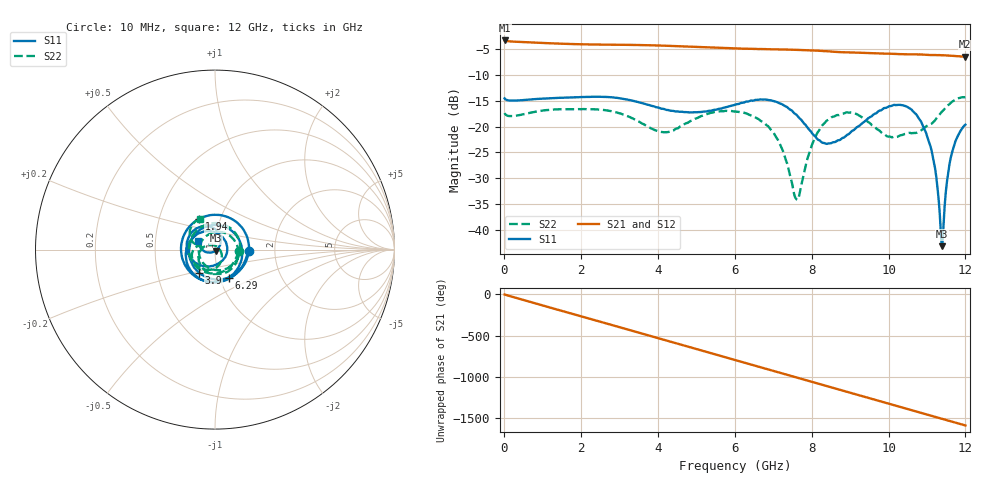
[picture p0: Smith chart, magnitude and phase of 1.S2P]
!Agilent Technologies,E5071C,MY46316741,A.11.02
!Date: Fri Apr 15 15:48:09 2022
!Data & Calibration Information:
!Freq	S11:SOLT2(ON)	S21:SOLT2(ON)	S12:SOLT2(ON)	S22:SOLT2(ON)
!PortZ  Port1:50+j0  Port2:50+j0
!Above PortZ is port z conversion or system Z0 setting when saving the data.
!When reading, reference impedance value at option line is always used.
# Hz S dB R 50
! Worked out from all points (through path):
!   1200 points, 10 MHz to 12 GHz, reference 50 ohm
!   highest |S21| = -3.32 dB at 10 MHz (marker M1); lowest = -6.5 dB at 11.99 GHz (marker M2)
!   group delay of S21, straight-line fit = 366 ps
!   lowest |S11| = -43.1 dB at 11.39 GHz (marker M3), VSWR 1.01, Z = 50.4 - j0.581 ohm
!   |S11| at or under -10 dB: start of sweep to end of sweep
!   |S22| runs from -34.2 to -14.3 dB; largest |S21 - S12| = 0.004
!   S11 on the Smith chart (normalised r, x): 10 MHz: 1.46, -0.03; 1.94 GHz: 0.79, +0.28; 3.9 GHz: 0.81, -0.22; 6.29 GHz: 1.11, -0.36; 12 GHz: 0.83, +0.08
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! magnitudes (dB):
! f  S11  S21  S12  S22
! 10 MHz  -14.5  -3.3  -3.3  -17.4
! 1.94 GHz  -14.3  -4.1  -4.0  -16.6
! 2.01 GHz  -14.3  -4.1  -4.1  -16.6
! 3.9 GHz  -16.1  -4.3  -4.3  -20.6
! 4.01 GHz  -16.3  -4.3  -4.3  -20.9
! 6.01 GHz  -15.7  -4.9  -4.9  -17.1
! 6.29 GHz  -15.2  -4.9  -4.9  -17.4
! 7.07 GHz  -15.2  -5.1  -5.0  -22.0
! 7.61 GHz  -17.7  -5.1  -5.1  -34.1
! 8.01 GHz  -21.3  -5.2  -5.2  -23.5
! 8.37 GHz  -23.3  -5.4  -5.4  -19.0
! 8.92 GHz  -21.6  -5.6  -5.6  -17.3
! 10.01 GHz  -16.1  -5.9  -5.9  -21.9
! 10.53 GHz  -16.4  -6.0  -6.0  -21.2
! 10.92 GHz  -20.3  -6.1  -6.1  -20.3
! 11.18 GHz  -26.8  -6.1  -6.1  -19.0
! 11.39 GHz  -43.1  -6.2  -6.2  -17.1
! 11.43 GHz  -39.1  -6.2  -6.2  -16.8
! 11.54 GHz  -29.6  -6.2  -6.2  -15.9
! 11.63 GHz  -25.6  -6.3  -6.3  -15.3
! 11.99 GHz  -19.7  -6.5  -6.4  -14.3
! 12 GHz  -19.6  -6.5  -6.4  -14.3
